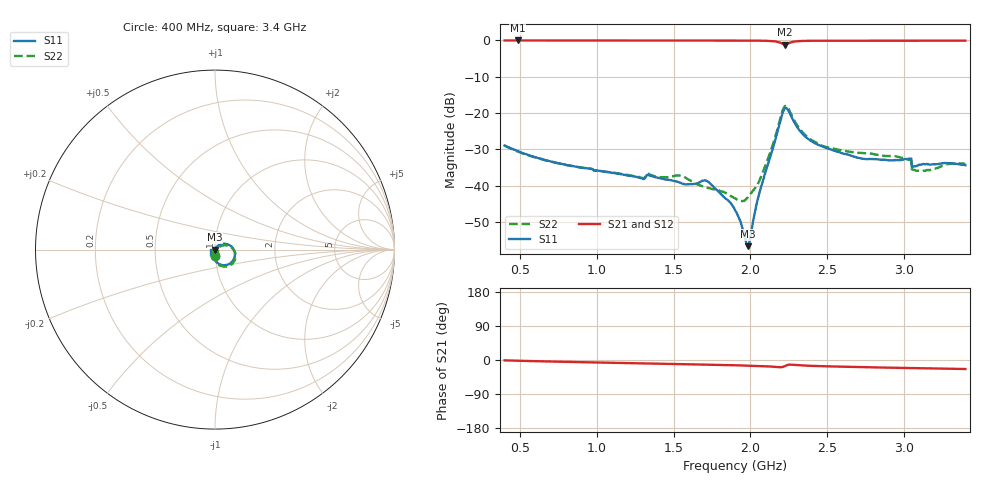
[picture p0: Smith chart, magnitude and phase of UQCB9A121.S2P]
!  Part Number  UQCB7A121	Mounting Orientation: Vertical
!  Description: RF capacitors
!  Application: Coupling, Bypass, Tuning, DC Block
!  Filters, Matching
# GHZ S DB R 50
! Freq  |S11|  S11 Ph  |S21|  S21 Ph  |S12|  S12 Ph  |S22|  S22 Ph
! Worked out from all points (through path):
!   801 points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, 400 MHz to 3.4 GHz, reference 50 ohm
!   highest |S21| = -0.01 dB at 486 MHz (marker M1); lowest = -1.1 dB at 2.226 GHz (marker M2)
!   group delay of S21, straight-line fit = 20.1 ps
!   lowest |S11| = -56.7 dB at 1.983 GHz (marker M3), VSWR 1.00, Z = 49.9 + j0.0549 ohm
!   |S11| at or under -10 dB: start of sweep to end of sweep
!   |S22| runs from -44.3 to -18.1 dB; largest |S21 - S12| = 0.0012
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0.4  -28.97 -89.9  -0.01 -1.0  -0.02 -1.0  -29.01 -90.0
0.486  -30.56 -90.7  -0.01 -1.9  -0.02 -1.9  -30.65 -90.2
0.903  -35.10 -95.0  -0.02 -5.8  -0.02 -5.8  -35.06 -90.2
1.401  -37.90 -103.9  -0.03 -9.7  -0.03 -9.7  -37.66 -83.6
1.548  -39.31 -106.9  -0.04 -10.9  -0.04 -10.9  -37.26 -85.5
1.713  -38.67 -112.5  -0.05 -12.3  -0.05 -12.3  -40.59 -80.6
1.9  -46.75 -131.9  -0.05 -13.9  -0.05 -13.9  -43.53 -54.0
1.949  -51.72 -149.1  -0.05 -14.4  -0.05 -14.4  -44.31 -31.9
1.983  -56.72 157.8  -0.05 -14.8  -0.05 -14.8  -43.30 -12.8
1.998  -54.82 118.8  -0.05 -14.9  -0.06 -14.9  -42.49 -5.7
2.031  -46.92 82.3  -0.06 -15.4  -0.07 -15.4  -40.67 7.2
2.073  -39.97 67.5  -0.08 -16.0  -0.09 -16.0  -37.25 24.9
2.185  -23.79 30.2  -0.48 -18.9  -0.48 -19.0  -23.03 19.2
2.226  -18.65 -21.0  -1.14 -15.6  -1.15 -15.6  -18.09 -26.6
2.331  -25.36 -93.1  -0.16 -14.2  -0.16 -14.3  -24.91 -90.4
2.403  -27.90 -101.5  -0.09 -15.5  -0.10 -15.5  -27.55 -95.4
2.706  -32.39 -111.7  -0.06 -18.6  -0.07 -18.6  -31.00 -97.9
2.901  -33.08 -108.2  -0.08 -20.2  -0.08 -20.2  -31.86 -103.2
3.033  -32.61 -107.3  -0.10 -21.1  -0.11 -21.2  -32.92 -112.4
3.066  -34.70 -108.7  -0.10 -21.4  -0.11 -21.4  -35.71 -93.8
3.089  -34.51 -109.1  -0.11 -21.5  -0.11 -21.5  -35.94 -91.3
3.4  -34.41 -134.1  -0.07 -23.8  -0.07 -23.8  -34.03 -89.7
